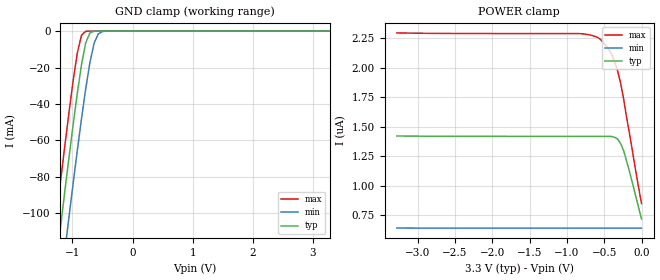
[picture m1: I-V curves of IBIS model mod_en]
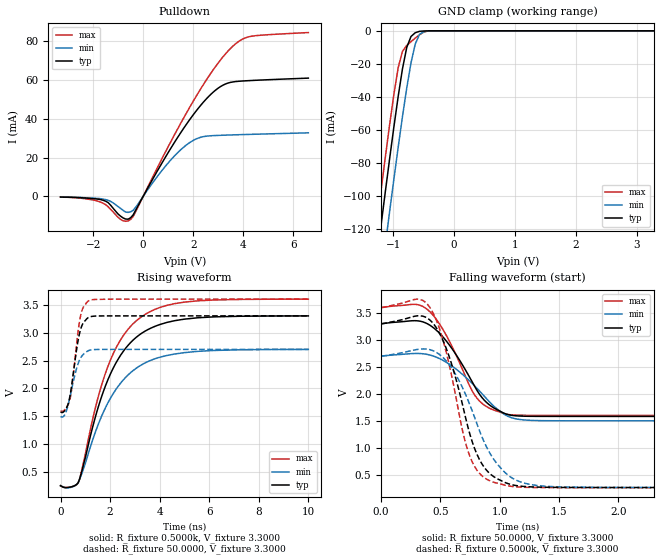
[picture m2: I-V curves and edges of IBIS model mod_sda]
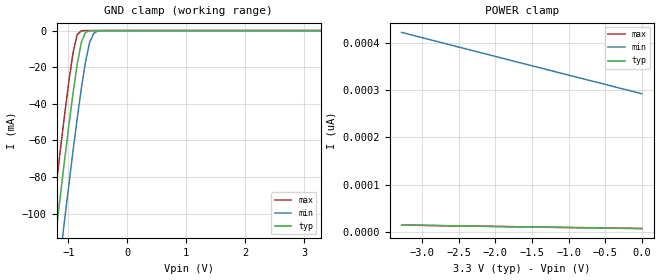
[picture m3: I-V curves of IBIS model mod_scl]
| IBIS (I/O, Buffer, Information, Specification) Model, officially
| electronic behavioral standard for Buffer structures of digital pins.
[IBIS ver]  4.0
[File name] m24c32_g5_tssop8.ibs
[File Rev]  1.0
[Date]   21 April 2015
[Source]   CAD & Design Services (Catania) - STMicroelectronics
[Notes]
   (Note1)  This IBIS model includes the TSSOP8 package data
   (Note2)  This IBIS model has some Notes about the non-monotonicity
   of the I-V curves, but they are not indicative of problems
   inside the model;
[Copyright] (c) 2015 STMicroelectronics
|   Component M24C32
[Component] M24C32
[Manufacturer] STMicroelectronics
[Package]
| variable   typ   min   max
R_pkg   0.0   0.0   0.0
L_pkg   0.0H   0.0H   0.0H
C_pkg   0.0F   0.0F   0.0F
[Pin]  signal_name   model_name   R_pin   L_pin   C_pin
1   E0   mod_en   NA   NA   NA
2   E1   mod_en   NA   NA   NA
3   E2   mod_en   NA   NA   NA
4   VSS   GND   NA   NA   NA
5   SDA   mod_sda   NA   NA   NA
6   SCL   mod_scl   NA   NA   NA
7   WCN   mod_wcn   NA   NA   NA
8   VCC   POWER   NA   NA   NA
[Package Model]  182696_TSSOP8
[Define Package Model]  182696_TSSOP8
[Manufacturer]  STMicroelectronics
[OEM]  STMicroelectronics
[Description]  8 pin TSSOP package
[Number Of Pins]  8
[Pin Numbers]
|Pin Num   Terminal Name
1   | net1
2   | net2
3   | net3
4   | net4_GND
5   | net5
6   | net6
7   | net7
8   | net8_VDD
[Model Data]
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[End Model Data]
[End Package Model]
| Models and submodels in the file (4): mod_en (Input), mod_sda (I/O_open_drain), mod_scl (Input), mod_wcn (Input)
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|   Model mod_en
[Model]   mod_en
Model_type Input
Vinl   =   1.000V
Vinh   =   2.300V
C_comp   2.119pF   2.023pF   2.323pF
[Temperature Range]  25.0000   0.1050k   -40.0000
[Voltage Range]   3.3000V   2.7000V   3.6000V
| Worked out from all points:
|   GND clamp passes 1 mA (typ) near -0.71 V on its own axis
[GND_clamp]
|Voltage   I(typ)   I(min)   I(max)
-3.3V     -716.1mA   -747.3mA   -693mA
-1.34V    -146.9mA   -179.9mA   -121.9mA
-1.27V    -127.3mA   -160.3mA   -102.2mA
-1.2V     -107.9mA   -140.9mA   -82.83mA
-1.13V    -88.69mA   -121.6mA   -63.73mA
-1.06V    -69.88mA   -102.6mA   -45.18mA
-920mV    -34.23mA   -65.73mA   -12.14mA
-850mV    -18.54mA   -48.2mA    -2.271mA
-780mV    -6.491mA   -31.8mA    -129.9uA
-640mV    -95.2uA    -6.689mA   -224.5nA
-500mV    -655.8nA   -240.8uA   -381.5pA
3.28V     6.871pA    315.5pA    6.69pA
[POWER_clamp]
|Voltage   I(typ)   I(min)   I(max)
-3.28V    1.421uA    642nA      2.294uA
-840mV    1.418uA    641nA      2.288uA
-680mV    1.418uA    641nA      2.275uA
-560mV    1.418uA    641nA      2.244uA
-480mV    1.418uA    641nA      2.189uA
-400mV    1.417uA    641nA      2.111uA
-320mV    1.395uA    641nA      1.97uA
-280mV    1.356uA    641nA      1.869uA
-240mV    1.298uA    640.9nA    1.735uA
-160mV    1.118uA    640.9nA    1.438uA
-80mV     918.4nA    640.9nA    1.133uA
0V        718.4nA    640.9nA    848.4nA
|   Model mod_sda
[Model]   mod_sda
Model_type I/O_open_drain
Polarity   Inverting
Vinl   =   1.000V
Vinh   =   2.300V
Vmeas  =   1.650V
Cref   =   10pF
Rref   =   1k
Vref   =   3.300V
C_comp   2.925pF   2.793pF   3.207pF
[Temperature Range]   25.0000   0.1050k   -40.0000
[Voltage Range]   3.3000V   2.7000V   3.6000V
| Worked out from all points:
|   slope of the pulldown table from 0 to 0.495 V, typ, clamps not added: 43.1 ohm
|   GND clamp passes 1 mA (typ) near -0.63 V on its own axis
|   rising waveform, R_fixture 0.5000k, V_fixture 3.3000: 20-80 % time 1.52ns typ, 1.59ns min, 1.46ns max; typ from 0.259 V to 3.3 V
|   rising waveform, R_fixture 50.0000, V_fixture 3.3000: 20-80 % time 348ps typ, 399ps min, 314ps max; typ from 1.58 V to 3.3 V
|   falling waveform, R_fixture 50.0000, V_fixture 3.3000: 20-80 % time 295ps typ, 336ps min, 263ps max; typ from 3.3 V to 1.58 V
|   falling waveform, R_fixture 0.5000k, V_fixture 3.3000: 20-80 % time 237ps typ, 297ps min, 205ps max; typ from 3.3 V to 0.259 V
[Pulldown]
|Voltage   I(typ)   I(min)   I(max)
-3.3V     -337uA     -229uA     -402.1uA
-1.6V     -1.974mA   -1.361mA   -3.521mA
-1.4V     -3.186mA   -1.987mA   -5.313mA
-900mV    -10.19mA   -6.185mA   -11.87mA
-500mV    -11.02mA   -7.93mA    -11.9mA
900mV     20.46mA    15.74mA    23.16mA
1.7V      36.68mA    26.26mA    42.35mA
2.1V      43.79mA    29.55mA    51.26mA
2.6V      51.34mA    31.18mA    61.55mA
3.4V      58.52mA    31.67mA    75.13mA
4.2V      59.72mA    31.98mA    82.29mA
6.6V      61.03mA    32.81mA    84.54mA
[GND_clamp]
|Voltage   I(typ)   I(min)   I(max)
-3.3V     -755.4mA   -785.4mA   -736.3mA
-1.27V    -137.4mA   -169.6mA   -116.3mA
-1.2V     -117mA     -149.2mA   -95.97mA
-1.13V    -96.84mA   -129mA     -75.94mA
-1.06V    -77.07mA   -109mA     -56.49mA
-920mV    -39.55mA   -70.31mA   -22.25mA
-850mV    -22.98mA   -51.9mA    -12.41mA
-780mV    -10.07mA   -34.64mA   -8.857mA
-640mV    -1.148mA   -7.967mA   -4.409mA
-570mV    -312.2uA   -2.174mA   -2.407mA
-430mV    -26.03uA   -157.9uA   -67.74uA
3.28V     145.8pA    1.447nA    140.6pA
[Ramp]
| variable   typ   min   max
dV/dt_r  1.0319/0.4084n   0.7033/0.4736n   1.2005/0.3607n
dV/dt_f  1.0319/0.3354n   0.7033/0.3689n   1.2005/0.2837n
R_load = 50.0000
[Rising Waveform]
R_fixture= 0.5000k
V_fixture= 3.3000
V_fixture_min= 2.7000   | new T=105 (min)
V_fixture_max= 3.6000
|time   V(typ)   V(min)   V(max)
0s        259mV      260.9mV    254.5mV
330ps     228.5mV    221.7mV    230.5mV
710ps     311mV      313.6mV    306.2mV
1.45ns    1.559V     1.272V     1.731V
1.91ns    2.154V     1.74V      2.393V
2.53ns    2.664V     2.152V     2.945V
3.23ns    2.976V     2.413V     3.272V
4.03ns    3.148V     2.562V     3.454V
4.99ns    3.241V     2.641V     3.546V
10ns      3.299V     2.699V     3.6V
[Rising Waveform]
R_fixture= 50.0000
V_fixture= 3.3000
V_fixture_min= 2.7000   | new T=105 (min)
V_fixture_max= 3.6000
|time   V(typ)   V(min)   V(max)
0s        1.58V      1.499V     1.599V
200ps     1.622V     1.556V     1.634V
300ps     1.714V     1.697V     1.704V
380ps     1.864V     1.848V     1.806V
480ps     2.156V     2.053V     2.097V
660ps     2.731V     2.376V     2.843V
800ps     3.044V     2.538V     3.281V
920ps     3.176V     2.611V     3.456V
1.16ns    3.278V     2.683V     3.575V
10ns      3.3V       2.7V       3.6V
[Falling Waveform]
R_fixture= 50.0000
V_fixture= 3.3000
V_fixture_min= 2.7000   | New T=105 C ( min )
V_fixture_max= 3.6000
|time   V(typ)   V(min)   V(max)
0s        3.3V       2.7V       3.6V
280ps     3.357V     2.748V     3.661V
390ps     3.3V       2.731V     3.565V
570ps     2.921V     2.556V     3V
750ps     2.293V     2.231V     2.129V
810ps     2.058V     2.098V     1.914V
930ps     1.767V     1.813V     1.716V
1.09ns    1.605V     1.564V     1.611V
1.49ns    1.581V     1.5V       1.6V
10ns      1.58V      1.499V     1.599V
[Falling Waveform]
R_fixture= 0.5000k
V_fixture= 3.3000   | New T=105C (min)
V_fixture_min= 2.7000
V_fixture_max= 3.6000
|time   V(typ)   V(min)   V(max)
0s        3.3V       2.7V       3.6V
310ps     3.448V     2.825V     3.757V
410ps     3.372V     2.82V      3.606V
570ps     2.716V     2.555V     2.581V
690ps     1.765V     2.097V     1.28V
770ps     1.098V     1.672V     728.3mV
890ps     579.6mV    1.01V      415.3mV
1.09ns    319.8mV    458.3mV    284.9mV
1.68ns    261.5mV    266.4mV    256.9mV
10ns      259mV      260.9mV    254.5mV
|   Model mod_scl
[Model]   mod_scl
Model_type Input
Vinl   =   1.000V
Vinh   =   2.300V
C_comp   2.119pF   2.023pF   2.323pF
[Temperature Range]   25.0000   0.1050k   -40.0000
[Voltage Range]   3.3000V   2.7000V   3.6000V
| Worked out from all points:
|   GND clamp passes 1 mA (typ) near -0.71 V on its own axis
[GND_clamp]
|Voltage   I(typ)   I(min)   I(max)
-3.3V     -716.1mA   -747.3mA   -693mA
-1.34V    -146.9mA   -179.9mA   -121.9mA
-1.27V    -127.3mA   -160.3mA   -102.2mA
-1.2V     -107.9mA   -140.9mA   -82.83mA
-1.13V    -88.69mA   -121.6mA   -63.73mA
-1.06V    -69.88mA   -102.6mA   -45.18mA
-920mV    -34.23mA   -65.73mA   -12.14mA
-850mV    -18.54mA   -48.2mA    -2.271mA
-780mV    -6.491mA   -31.8mA    -129.9uA
-640mV    -95.2uA    -6.689mA   -224.5nA
-500mV    -655.8nA   -240.8uA   -381.5pA
3.28V     6.871pA    315.5pA    6.69pA
[POWER_clamp]
|Voltage   I(typ)   I(min)   I(max)
-3.28V    14.67pA    422.5pA    14.54pA
-2.52V    12.77pA    392.2pA    12.82pA
-1.44V    10.18pA    349.4pA    10.44pA
0V        6.915pA    292.7pA    7.361pA
